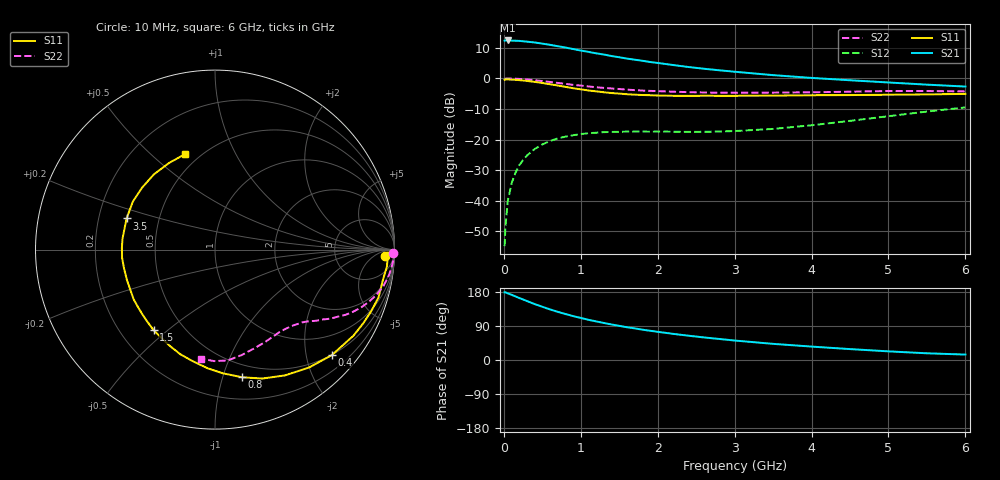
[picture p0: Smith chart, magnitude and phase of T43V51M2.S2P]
! Infineon Technologies  Discrete & RF Semiconductors
! BFR182T
! Si NPN RF Bipolar Junction Transistor in SC75
! VCE = 3.5 V  IC = 1.2 mA
! Common Emitter S-Parameters:  October  1999
# GHz  S  MA  R  50
!  f  S11  S21  S12  S22
! GHz  MAG  ANG  MAG  ANG  MAG  ANG  MAG  ANG
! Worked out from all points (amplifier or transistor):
!   36 points, 10 MHz to 6 GHz, reference 50 ohm
!   highest |S21| = 12.4 dB at 50 MHz (marker M1)
!   |S21| within 3 dB of that: start of sweep to 938.5 MHz
!   unconditionally stable (mu >= 1): 2.305 GHz to 4.506 GHz
!   at 250 MHz: K = 0.10, MSG = 19.4 dB, |S12| = -26.7 dB
!   at 1.4 GHz: K = 0.62, MSG = 12.4 dB, |S12| = -17.5 dB
!   at 6 GHz: K = 0.83, MSG = 3.4 dB, |S12| = -9.5 dB
!   S11 on the Smith chart (normalised r, x): 10 MHz: 25, -18; 400 MHz: 0.49, -2.52; 800 MHz: 0.38, -1.16; 1.5 GHz: 0.34, -0.45; 3.5 GHz: 0.32, +0.15; 6 GHz: 0.42, +0.65
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0.01  0.9495 -2.2  4.147 178.6  0.0018 85.7  0.9909 -1.2
0.02  0.9644 -0.9  4.17 178.7  0.0036 90.1  0.9911 -0.7
0.05  0.9625 -5.6  4.173 175.9  0.0097 86.7  0.9967 -2.1
0.1  0.9505 -10.4  4.149 172.2  0.019 85.4  0.9928 -4.2
0.2  0.9358 -21.4  4.107 163.6  0.0378 78.2  0.9796 -8.3
0.3  0.9086 -31.8  3.989 155.6  0.0546 72.1  0.9601 -12.2
0.4  0.8774 -42.0  3.868 147.6  0.0699 66.5  0.9331 -15.8
0.5  0.8405 -51.4  3.705 140.5  0.0829 60.9  0.904 -18.9
0.6  0.8018 -61.0  3.538 133.5  0.0946 56.4  0.8735 -21.8
0.7  0.7649 -69.9  3.363 127.2  0.1043 52.5  0.8427 -24.3
0.8  0.7273 -78.0  3.196 121.4  0.1113 49.1  0.8137 -26.5
0.9  0.69 -86.5  3.02 115.9  0.1175 45.7  0.7845 -28.3
1.1  0.634 -101.3  2.715 106.0  0.1269 40.9  0.7378 -31.6
1.3  0.593 -115.0  2.457 97.7  0.1321 37.1  0.6986 -34.3
1.5  0.564 -127.3  2.217 90.1  0.1338 34.8  0.6698 -36.5
1.8  0.5345 -144.1  1.943 80.0  0.1353 32.8  0.6321 -40.0
2.2  0.519 -161.1  1.654 69.0  0.1343 33.5  0.6061 -44.3
2.8  0.5189 178.9  1.357 55.5  0.1349 38.8  0.583 -52.2
3.5  0.5223 160.6  1.13 42.6  0.149 48.8  0.5856 -61.4
4.5  0.5332 139.6  0.932 28.8  0.2019 58.6  0.606 -75.8
5.5  0.5465 117.7  0.79 17.7  0.2867 59.3  0.6214 -90.4
6  0.5579 107.2  0.735 14.3  0.3354 56.7  0.6126 -97.1
